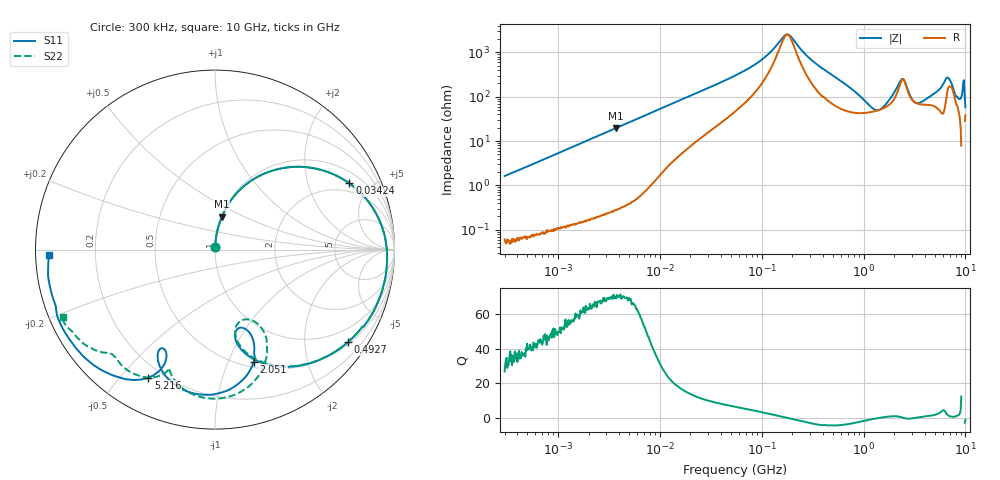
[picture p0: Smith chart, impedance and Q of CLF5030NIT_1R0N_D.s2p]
! S-Parameter Data Generated by TDK Corporation
! Copyright(C) 2019 TDK Corporation.
! All Rights Reserved.
! TDK P/N: CLF5030NIT-1R0N-D (Inductor)
! Property: L=1uH at 100kHz
! Size(LxWxT): 5.3x5x2.7mm
! Model Type: s2p (Touchstone File Format Version 1.0)
! Frequency: DC=Yes Start=0.3MHz Stop=10000MHz 802points Log-sweep
! Model Generated on May 10, 2019
! Port Assignments:
!  1 ---@@@--- 2
! Applicable Conditions:
!  Temperature = 25 degC
!  DC Bias Current = 0 A
!  Small Signal Operation
! Terms and conditions regarding TDK Simulation Models
! (1)This simulation model is being provided solely for informational purposes. Please refer to the specifications of the products in terms of detailed characteristics of such products.
! (2)In no event shall TDK Corporation of any of its subsidiaries be liable for any loss or damage arising, directly or indirectly,
!  From any information contained in this simulation model, including, but not limited to loss or damages arising from any inaccuracies, omissions or errors in connection with such information.
! (3)Any and all copyrights on this simulation model are owned by TDK Corporation.
!  Duplication or redistribution of this simulation model without prior written permission from TDK Corporation is prohibited.
! (4)This simulation model is subject to any modification or change without any prior notice.
! (5)Neither TDK Corporation nor any of its subsidiaries shall make any warranty, express or implied,
!  Including but not limited to the correctness, implied warranties of merchantability and fitness for a particular purpose with respect to this simulation models.
! (6)The use of this simulation model shall be deemed to have consented to the terms and conditions hereof.
# Hz S MA R 50
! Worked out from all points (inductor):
!   801 points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, 300 kHz to 10 GHz, reference 50 ohm
!   read as one part in series: L = 852 nH near 318.3 kHz
!   highest Q = 70.4 at 3.688 MHz (marker M1), where L = 833 nH
!   self-resonance near 178.5 MHz
!   S11 on the Smith chart (normalised r, x): 300 kHz: 1.00, +0.03; 34.24 MHz: 1.52, +3.71; 492.7 MHz: 0.56, -3.10; 2.051 GHz: 0.56, -1.24; 5.216 GHz: 0.15, -0.60; 10 GHz: 0.04, -0.02
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300000  0.01623 87.3  0.9991 -0.9  0.9991 -0.9  0.01638 87.8
1713600  0.08896 83.9  0.9945 -5.2  0.9946 -5.2  0.089 83.9
3688026  0.1879 78.2  0.9794 -11.0  0.9795 -11.0  0.1879 78.2
9671944  0.4473 61.3  0.8809 -26.9  0.881 -26.9  0.4472 61.3
3.424315e7  0.835 26.2  0.4659 -57.4  0.466 -57.4  0.8349 26.2
5.477226e7  0.9062 15.4  0.3051 -65.7  0.3052 -65.7  0.9062 15.4
1.00316e8  0.9506 3.7  0.1394 -69.5  0.1394 -69.5  0.9506 3.7
1.765741e8  0.9619 -6.9  0.03789 -10.4  0.03791 -10.4  0.962 -6.8
3.126428e8  0.9499 -20.2  0.1409 53.1  0.1409 53.1  0.9502 -20.1
4.926597e8  0.9024 -34.8  0.2715 43.1  0.2715 43.1  0.9032 -34.6
7.84152e8  0.7859 -55.9  0.4379 19.2  0.438 19.2  0.7863 -55.5
1.149233e9  0.5955 -74.2  0.5588 -12.9  0.5591 -12.9  0.5888 -73.8
1.767019e9  0.4939 -67.7  0.5136 -68.0  0.5137 -68.1  0.4511 -61.8
2.051294e9  0.6609 -70.9  0.3662 -91.7  0.3662 -91.8  0.6219 -62.2
2.446702e9  0.8104 -92.9  0.1707 -79.5  0.1706 -79.5  0.8203 -83.5
2.924554e9  0.7388 -113.4  0.2707 -66.1  0.271 -66.1  0.7908 -103.6
3.874538e9  0.6249 -116.4  0.3052 -111.3  0.3056 -111.4  0.7136 -111.2
5.21579e9  0.8033 -117.5  0.1692 -165.1  0.1696 -165.3  0.8233 -122.0
6.737565e9  0.933 -136.2  0.04654 -176.0  0.04564 -176.4  0.841 -137.0
8.322921e9  0.9415 -161.5  0.03881 171.4  0.03924 171.7  0.9237 -151.3
9.440974e9  0.9364 -173.2  0.008432 110.6  0.00841 110.2  0.9294 -156.5
1e10  0.9268 -178.0  0.01402 -42.2  0.01388 -42.1  0.9249 -156.1
